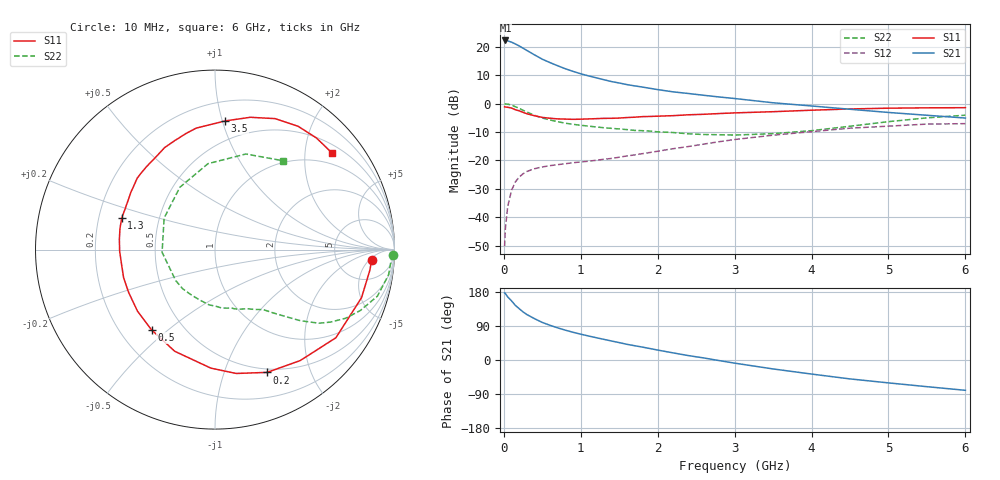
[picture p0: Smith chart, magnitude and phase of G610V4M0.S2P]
! SIEMENS Small Signal Semiconductors
! BFG193
! Si NPN RF Bipolar Junction Transistor in SOT223
! VCE = 10 V  IC = 4 mA
! Common Emitter S-Parameters:  August  1996
# GHz  S  MA  R  50
!  f  S11  S21  S12  S22
! GHz  MAG  ANG  MAG  ANG  MAG  ANG  MAG  ANG
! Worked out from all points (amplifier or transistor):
!   36 points, 10 MHz to 6 GHz, reference 50 ohm
!   highest |S21| = 22.2 dB at 20 MHz (marker M1)
!   |S21| within 3 dB of that: start of sweep to 267 MHz
!   unconditionally stable (mu >= 1): 1.227 GHz to 2.52 GHz
!   at 250 MHz: K = 0.28, MSG = 22.1 dB, |S12| = -24.7 dB
!   at 1.4 GHz: K = 1.08, MAG = 11.8 dB, |S12| = -19.3 dB
!   at 6 GHz: K = 0.87, MSG = 1.0 dB, |S12| = -7.1 dB
!   S11 on the Smith chart (normalised r, x): 10 MHz: 12, -6; 200 MHz: 0.46, -1.41; 500 MHz: 0.33, -0.44; 1.3 GHz: 0.30, +0.15; 3.5 GHz: 0.34, +1.02; 6 GHz: 0.70, +2.64
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0.01  0.8749 -3.7  12.75 177.1  0.0031 90.7  0.9917 -1.7
0.02  0.8704 -7.6  12.87 175.4  0.0063 83.7  0.9834 -3.4
0.05  0.8592 -18.2  12.65 166.6  0.0154 79.7  0.9771 -8.3
0.1  0.8336 -36.1  12.01 156.1  0.0298 72.0  0.9413 -16.0
0.15  0.7795 -52.5  11.16 144.0  0.0419 62.8  0.8783 -22.7
0.2  0.7432 -67.0  10.3 135.4  0.051 57.0  0.8225 -27.7
0.25  0.7001 -80.3  9.399 126.9  0.0582 51.7  0.7601 -32.1
0.3  0.6608 -92.0  8.575 119.9  0.064 47.9  0.7096 -35.3
0.4  0.6093 -111.6  7.16 108.9  0.0714 41.8  0.6189 -39.8
0.5  0.5702 -128.3  6.023 99.1  0.0767 38.0  0.5566 -42.7
0.6  0.5513 -141.6  5.248 91.6  0.0808 36.3  0.5139 -45.1
0.7  0.5371 -153.5  4.62 84.8  0.0842 35.2  0.4795 -47.4
0.9  0.527 -171.6  3.676 73.1  0.0911 34.5  0.4304 -51.1
1.1  0.5359 173.9  3.065 63.4  0.0968 35.1  0.4006 -56.4
1.3  0.5486 161.3  2.626 54.5  0.1048 36.1  0.3752 -61.4
1.6  0.567 145.8  2.154 41.4  0.1196 36.7  0.3481 -71.5
2.2  0.6121 122.6  1.605 18.8  0.1604 34.7  0.3093 -96.4
2.8  0.6668 104.0  1.304 -1.6  0.2132 27.5  0.2828 -129.4
3.5  0.719 85.5  1.031 -23.6  0.2776 13.4  0.2952 -177.1
4.5  0.8031 65.3  0.793 -49.9  0.3687 -7.6  0.3987 119.4
5.5  0.8404 47.7  0.622 -70.4  0.4351 -34.6  0.5597 72.1
6  0.8458 39.3  0.556 -80.0  0.4429 -49.9  0.6244 52.4
